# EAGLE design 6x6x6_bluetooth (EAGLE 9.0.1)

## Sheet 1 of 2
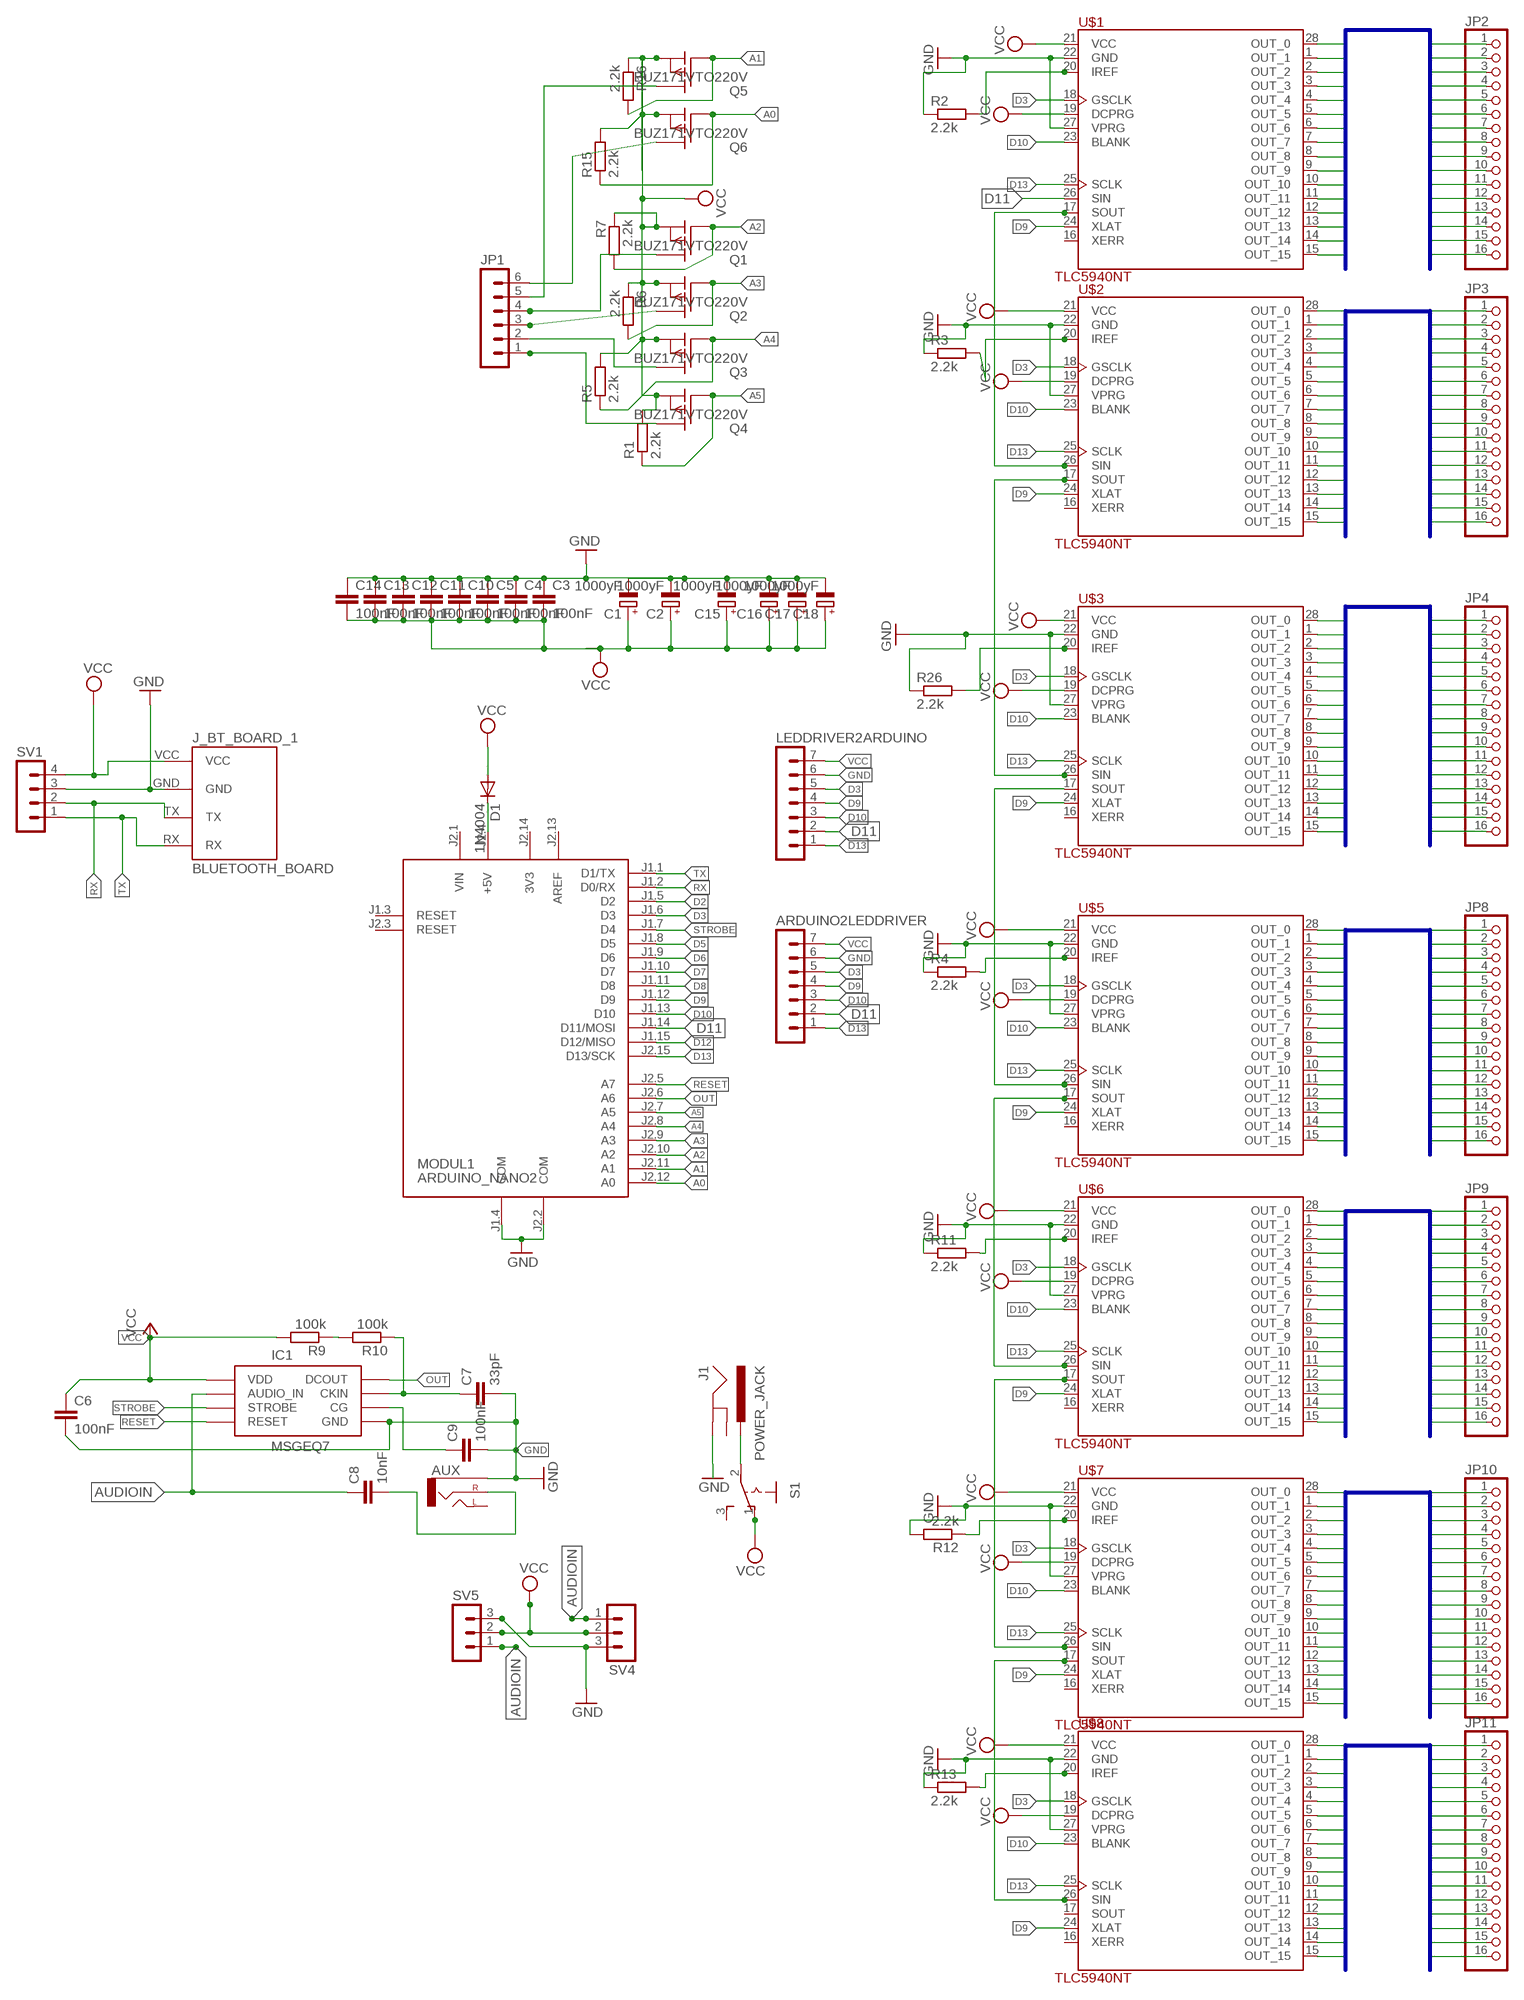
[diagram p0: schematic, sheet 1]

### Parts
ARDUINO2LEDDRIVER  MA07-1  [MA07-1]
AUX  AUDIO-JACKPTH  [AUDIO-JACK]
C1  1000yF  CPOL-EUE2.5-6  [E2,5-6]
C2  1000yF  CPOL-EUE2.5-6  [E2,5-6]
C3  100nF  C-EU025-024X044  [C025-024X044]
C4  100nF  C-EU025-024X044  [C025-024X044]
C5  100nF  C-EU025-024X044  [C025-024X044]
C6  100nF  C-EU025-025X050  [C025-025X050]
C7  33pF  C-EU025-025X050  [C025-025X050]
C8  10nF  C-EU025-025X050  [C025-025X050]
C9  100nF  C-EU025-025X050  [C025-025X050]
C10  100nF  C-EU025-024X044  [C025-024X044]
C11  100nF  C-EU025-024X044  [C025-024X044]
C12  100nF  C-EU025-024X044  [C025-024X044]
C13  100nF  C-EU025-024X044  [C025-024X044]
C14  100nF  C-EU025-024X044  [C025-024X044]
C15  1000yF  CPOL-EUE2.5-6  [E2,5-6]
C16  1000yF  CPOL-EUE2.5-6  [E2,5-6]
C17  1000yF  CPOL-EUE2.5-6  [E2,5-6]
C18  1000yF  CPOL-EUE2.5-6  [E2,5-6]
D1  1N4004  [DO41-10]
IC1  MSGEQ7DIP  [DIL08]
J1  POWER_JACK  [POWER_JACK_PTH]
J_BT_BOARD_1  BLUETOOTH_BOARD  [BT_BOARD_FOOTPRINT]
JP1  MA06-1  [MA06-1]
JP2  PINHD-1X16  [1X16]
JP3  PINHD-1X16  [1X16]
JP4  PINHD-1X16  [1X16]
JP8  PINHD-1X16  [1X16]
JP9  PINHD-1X16  [1X16]
JP10  PINHD-1X16  [1X16]
JP11  PINHD-1X16  [1X16]
LEDDRIVER2ARDUINO  MA07-1  [MA07-1]
MODUL1  ARDUINO_NANO2  [ARDUINO_NANO2]
Q1  BUZ171VTO220V  [TO220V]
Q2  BUZ171VTO220V  [TO220V]
Q3  BUZ171VTO220V  [TO220V]
Q4  BUZ171VTO220V  [TO220V]
Q5  BUZ171VTO220V  [TO220V]
Q6  BUZ171VTO220V  [TO220V]
R1  2.2k  R-EU_0204/7  [0204/7]
R2  2.2k  R-EU_0207/10  [0207/10]
R3  2.2k  R-EU_0207/10  [0207/10]
R4  2.2k  R-EU_0204/7  [0204/7]
R5  2.2k  R-EU_0204/7  [0204/7]
R6  2.2k  R-EU_0204/7  [0204/7]
R7  2.2k  R-EU_0204/7  [0204/7]
R9  100k  R-EU_0204/2V  [0204V]
R10  100k  R-EU_0204/2V  [0204V]
R11  2.2k  R-EU_0204/2V  [0204V]
R12  2.2k  R-EU_0204/2V  [0204V]
R13  2.2k  R-EU_0204/2V  [0204V]
R15  2.2k  R-EU_0204/7  [0204/7]
R16  2.2k  R-EU_0204/7  [0204/7]
R26  2.2k  R-EU_0204/5  [0204/5]
S1  255SB  [255SB]
SV1  MA04-1  [MA04-1]
SV4  MA03-1  [MA03-1]
SV5  MA03-1  [MA03-1]
U$1  TLC5940NT  [DIP-28]
U$2  TLC5940NT  [DIP-28]
U$3  TLC5940NT  [DIP-28]
U$5  TLC5940NT  [DIP-28]
U$6  TLC5940NT  [DIP-28]
U$7  TLC5940NT  [DIP-28]
U$8  TLC5940NT  [DIP-28]

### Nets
A0: MODUL1.J2.12(A0) Q6.1(G) R15.1
A1: MODUL1.J2.11(A1) Q5.1(G) R16.2
A2: MODUL1.J2.10(A2) Q1.1(G) R7.2
A3: MODUL1.J2.9(A3) Q2.1(G) R6.2
A4: MODUL1.J2.8(A4) Q3.1(G) R5.1
A5: MODUL1.J2.7(A5) Q4.1(G) R1.1
AUDIOIN: C8.1 IC1.5(AUDIO_IN) SV4.1 SV5.1
D2: MODUL1.J1.5(D2)
D3: ARDUINO2LEDDRIVER.5 LEDDRIVER2ARDUINO.5 MODUL1.J1.6(D3) U$1.18(GSCLK) U$2.18(GSCLK) U$3.18(GSCLK) U$5.18(GSCLK) U$6.18(GSCLK) U$7.18(GSCLK) U$8.18(GSCLK)
D5: MODUL1.J1.8(D5)
D6: MODUL1.J1.9(D6)
D7: MODUL1.J1.10(D7)
D8: MODUL1.J1.11(D8)
D9: ARDUINO2LEDDRIVER.4 LEDDRIVER2ARDUINO.4 MODUL1.J1.12(D9) U$1.24(XLAT) U$2.24(XLAT) U$3.24(XLAT) U$5.24(XLAT) U$6.24(XLAT) U$7.24(XLAT) U$8.24(XLAT)
D10: ARDUINO2LEDDRIVER.3 LEDDRIVER2ARDUINO.3 MODUL1.J1.13(D10) U$1.23(BLANK) U$2.23(BLANK) U$3.23(BLANK) U$5.23(BLANK) U$6.23(BLANK) U$7.23(BLANK) U$8.23(BLANK)
D11: ARDUINO2LEDDRIVER.2 LEDDRIVER2ARDUINO.2 MODUL1.J1.14(D11/MOSI) U$1.26(SIN)
D12: MODUL1.J1.15(D12/MISO)
D13: ARDUINO2LEDDRIVER.1 LEDDRIVER2ARDUINO.1 MODUL1.J2.15(D13/SCK) U$1.25(SCLK) U$2.25(SCLK) U$3.25(SCLK) U$5.25(SCLK) U$6.25(SCLK) U$7.25(SCLK) U$8.25(SCLK)
GND: ARDUINO2LEDDRIVER.6 AUX.SLEEVE C1.- C2.- C3.1 C4.1 C5.1 C6.2 C7.2 C9.2 C10.1 C11.1 C12.1 C13.1 C14.1 C15.- C16.- C17.- C18.- IC1.2(GND) J1.GND J_BT_BOARD_1.GND LEDDRIVER2ARDUINO.6 MODUL1.J1.4(COM) MODUL1.J2.2(COM) R2.1 R3.1 R4.1 R11.1 R12.2 R13.1 R26.1 SV1.3 SV4.3 SV5.3 U$1.22(GND) U$1.27(VPRG) U$2.22(GND) U$2.27(VPRG) U$3.22(GND) U$3.27(VPRG) U$5.22(GND) U$5.27(VPRG) U$6.22(GND) U$6.27(VPRG) U$7.22(GND) U$7.27(VPRG) U$8.22(GND) U$8.27(VPRG)
N$1: J1.PWR S1.2(P)
N$2: JP1.3 Q2.2(D)
N$4: JP1.1 Q4.2(D)
N$5: U$1.17(SOUT) U$2.26(SIN)
N$6: U$2.17(SOUT) U$3.26(SIN)
N$7: R26.2 U$3.20(IREF)
N$8: R3.2 U$2.20(IREF)
N$9: R2.2 U$1.20(IREF)
N$10: JP1.2 Q3.2(D)
N$11: JP1.4 Q1.2(D)
N$55: AUX.RING(RIGHT) C8.2
N$93: C9.1 IC1.6(CG)
N$94: C7.1 IC1.8(CKIN) R10.1
N$95: R9.1 R10.2
N$96: U$3.17(SOUT) U$5.26(SIN)
N$97: JP1.5 Q5.2(D)
N$98: R4.2 U$5.20(IREF)
N$99: U$5.17(SOUT) U$6.26(SIN)
N$100: U$6.17(SOUT) U$7.26(SIN)
N$101: R11.2 U$6.20(IREF)
N$102: D1.C MODUL1.J2.4(+5V)
N$103: U$7.17(SOUT) U$8.26(SIN)
N$104: R12.1 U$7.20(IREF)
N$105: JP1.6 Q6.2(D)
N$107: R13.2 U$8.20(IREF)
OUT: IC1.3(DCOUT) MODUL1.J2.6(A6)
RESET: IC1.7(RESET) MODUL1.J2.5(A7)
RX: J_BT_BOARD_1.TX MODUL1.J1.2(D0/RX) SV1.2
STROBE: IC1.4(STROBE) MODUL1.J1.7(D4)
T1OUT0: JP2.1 U$1.28(OUT_0)
T1OUT1: JP2.2 U$1.1(OUT_1)
T1OUT2: JP2.3 U$1.2(OUT_2)
T1OUT3: JP2.4 U$1.3(OUT_3)
T1OUT4: JP2.5 U$1.4(OUT_4)
T1OUT5: JP2.6 U$1.5(OUT_5)
T1OUT6: JP2.7 U$1.6(OUT_6)
T1OUT7: JP2.8 U$1.7(OUT_7)
T1OUT8: JP2.9 U$1.8(OUT_8)
T1OUT9: JP2.10 U$1.9(OUT_9)
T1OUT10: JP2.11 U$1.10(OUT_10)
T1OUT11: JP2.12 U$1.11(OUT_11)
T1OUT12: JP2.13 U$1.12(OUT_12)
T1OUT13: JP2.14 U$1.13(OUT_13)
T1OUT14: JP2.15 U$1.14(OUT_14)
T1OUT15: JP2.16 U$1.15(OUT_15)
T2OUT0: JP3.1 U$2.28(OUT_0)
T2OUT1: JP3.2 U$2.1(OUT_1)
T2OUT2: JP3.3 U$2.2(OUT_2)
T2OUT3: JP3.4 U$2.3(OUT_3)
T2OUT4: JP3.5 U$2.4(OUT_4)
T2OUT5: JP3.6 U$2.5(OUT_5)
T2OUT6: JP3.7 U$2.6(OUT_6)
T2OUT7: JP3.8 U$2.7(OUT_7)
T2OUT8: JP3.9 U$2.8(OUT_8)
T2OUT9: JP3.10 U$2.9(OUT_9)
T2OUT10: JP3.11 U$2.10(OUT_10)
T2OUT11: JP3.12 U$2.11(OUT_11)
T2OUT12: JP3.13 U$2.12(OUT_12)
T2OUT13: JP3.14 U$2.13(OUT_13)
T2OUT14: JP3.15 U$2.14(OUT_14)
T2OUT15: JP3.16 U$2.15(OUT_15)
T3OUT_0: JP4.1 U$3.28(OUT_0)
T3OUT_1: JP4.2 U$3.1(OUT_1)
T3OUT_2: JP4.3 U$3.2(OUT_2)
T3OUT_3: JP4.4 U$3.3(OUT_3)
T3OUT_4: JP4.5 U$3.4(OUT_4)
T3OUT_5: JP4.6 U$3.5(OUT_5)
T3OUT_6: JP4.7 U$3.6(OUT_6)
T3OUT_7: JP4.8 U$3.7(OUT_7)
T3OUT_8: JP4.9 U$3.8(OUT_8)
T3OUT_9: JP4.10 U$3.9(OUT_9)
T3OUT_10: JP4.11 U$3.10(OUT_10)
T3OUT_11: JP4.12 U$3.11(OUT_11)
T3OUT_12: JP4.13 U$3.12(OUT_12)
T3OUT_13: JP4.14 U$3.13(OUT_13)
T3OUT_14: JP4.15 U$3.14(OUT_14)
T3OUT_15: JP4.16 U$3.15(OUT_15)
T4OUT0: JP8.1 U$5.28(OUT_0)
T4OUT1: JP8.2 U$5.1(OUT_1)
T4OUT2: JP8.3 U$5.2(OUT_2)
T4OUT3: JP8.4 U$5.3(OUT_3)
T4OUT4: JP8.5 U$5.4(OUT_4)
T4OUT5: JP8.6 U$5.5(OUT_5)
T4OUT6: JP8.7 U$5.6(OUT_6)
T4OUT7: JP8.8 U$5.7(OUT_7)
T4OUT8: JP8.9 U$5.8(OUT_8)
T4OUT9: JP8.10 U$5.9(OUT_9)
T4OUT10: JP8.11 U$5.10(OUT_10)
T4OUT11: JP8.12 U$5.11(OUT_11)
T4OUT12: JP8.13 U$5.12(OUT_12)
T4OUT13: JP8.14 U$5.13(OUT_13)
T4OUT14: JP8.15 U$5.14(OUT_14)
T4OUT15: JP8.16 U$5.15(OUT_15)
T5OUT0: JP9.1 U$6.28(OUT_0)
T5OUT1: JP9.2 U$6.1(OUT_1)
T5OUT2: JP9.3 U$6.2(OUT_2)
T5OUT3: JP9.4 U$6.3(OUT_3)
T5OUT4: JP9.5 U$6.4(OUT_4)
T5OUT5: JP9.6 U$6.5(OUT_5)
T5OUT6: JP9.7 U$6.6(OUT_6)
T5OUT7: JP9.8 U$6.7(OUT_7)
T5OUT8: JP9.9 U$6.8(OUT_8)
T5OUT9: JP9.10 U$6.9(OUT_9)
T5OUT10: JP9.11 U$6.10(OUT_10)
T5OUT11: JP9.12 U$6.11(OUT_11)
T5OUT12: JP9.13 U$6.12(OUT_12)
T5OUT13: JP9.14 U$6.13(OUT_13)
T5OUT14: JP9.15 U$6.14(OUT_14)
T5OUT15: JP9.16 U$6.15(OUT_15)
T6OUT0: JP10.1 U$7.28(OUT_0)
T6OUT1: JP10.2 U$7.1(OUT_1)
T6OUT2: JP10.3 U$7.2(OUT_2)
T6OUT3: JP10.4 U$7.3(OUT_3)
T6OUT4: JP10.5 U$7.4(OUT_4)
T6OUT5: JP10.6 U$7.5(OUT_5)
T6OUT6: JP10.7 U$7.6(OUT_6)
T6OUT7: JP10.8 U$7.7(OUT_7)
T6OUT8: JP10.9 U$7.8(OUT_8)
T6OUT9: JP10.10 U$7.9(OUT_9)
T6OUT10: JP10.11 U$7.10(OUT_10)
T6OUT11: JP10.12 U$7.11(OUT_11)
T6OUT12: JP10.13 U$7.12(OUT_12)
T6OUT13: JP10.14 U$7.13(OUT_13)
T6OUT14: JP10.15 U$7.14(OUT_14)
T6OUT15: JP10.16 U$7.15(OUT_15)
T7OUT0: JP11.1 U$8.28(OUT_0)
T7OUT1: JP11.2 U$8.1(OUT_1)
T7OUT2: JP11.3 U$8.2(OUT_2)
T7OUT3: JP11.4 U$8.3(OUT_3)
T7OUT4: JP11.5 U$8.4(OUT_4)
T7OUT5: JP11.6 U$8.5(OUT_5)
T7OUT6: JP11.7 U$8.6(OUT_6)
T7OUT7: JP11.8 U$8.7(OUT_7)
T7OUT8: JP11.9 U$8.8(OUT_8)
T7OUT9: JP11.10 U$8.9(OUT_9)
T7OUT10: JP11.11 U$8.10(OUT_10)
T7OUT11: JP11.12 U$8.11(OUT_11)
T7OUT12: JP11.13 U$8.12(OUT_12)
T7OUT13: JP11.14 U$8.13(OUT_13)
T7OUT14: JP11.15 U$8.14(OUT_14)
T7OUT15: JP11.16 U$8.15(OUT_15)
TX: J_BT_BOARD_1.RX MODUL1.J1.1(D1/TX) SV1.1
VCC: ARDUINO2LEDDRIVER.7 C1.+ C2.+ C3.2 C4.2 C5.2 C6.1 C10.2 C11.2 C12.2 C13.2 C14.2 C15.+ C16.+ C17.+ C18.+ D1.A IC1.1(VDD) J_BT_BOARD_1.VCC LEDDRIVER2ARDUINO.7 Q1.3(S) Q2.3(S) Q3.3(S) Q4.3(S) Q5.3(S) Q6.3(S) R1.2 R5.2 R6.1 R7.1 R9.2 R15.2 R16.1 S1.1(O) SV1.4 SV4.2 SV5.2 U$1.19(DCPRG) U$1.21(VCC) U$2.19(DCPRG) U$2.21(VCC) U$3.19(DCPRG) U$3.21(VCC) U$5.19(DCPRG) U$6.19(DCPRG) U$6.21(VCC) U$7.19(DCPRG) U$7.21(VCC) U$8.19(DCPRG) U$8.21(VCC)
Unconnected: AUX.TIP(LEFT) J1.GNDBREAK MODUL1.J1.3(RESET) MODUL1.J2.3(RESET) S1.3(S) U$1.16(XERR) U$2.16(XERR) U$3.16(XERR) U$5.16(XERR) U$6.16(XERR) U$7.16(XERR) U$8.16(XERR) U$8.17(SOUT)

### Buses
T3OUT_[0..15]
T2OUT[0..15]
T1OUT[0..15]
T4OUT[0..15]
T5OUT[0..15]
T6OUT[0..15]
T7OUT[0..15]

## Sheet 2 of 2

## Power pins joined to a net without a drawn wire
3V3: MODUL1.J2.14(3V3)
AREF: MODUL1.J2.13(AREF)
VCC: U$5.21(VCC)
VIN: MODUL1.J2.1(VIN)

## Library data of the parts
ARDUINO2LEDDRIVER LEDDRIVER2ARDUINO = con-lstb:MA07-1: PIN HEADER; OC_FARNELL: unknown; OC_NEWARK: unknown
AUX = connector:AUDIO-JACK: 3.5mm Audio Jack Simple 3.5mm common PCB mount audio jack.; DIGIKEY: CP1-3524N-ND
C1 C2 C15-C18 = resistor:CPOL-EU: POLARIZED CAPACITOR, European symbol
C3-C14 = resistor:C-EU: CAPACITOR, European symbol
D1 = diode:1N4004: DIODE
IC1 = msgeq7:MSGEQ7: 7-band graphic equalizer
J1 = SparkFun-Connectors:POWER_JACK: Power Jack Connector This is the standard 5.5mm barrel jack for power. The PTH is the most common, proven, reliable, footprint. The Slot footprint only works if the mill layer is transmitted to the PCB fab house so be warned. Here are the connectors we sell at SparkFun: DC Barrel Power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; PROD_ID: CONN-08197
J_BT_BOARD_1 = Bluetooth HC-05:BLUETOOTH_BOARD: Bluetooth Board V1.05
JP1 = con-lstb:MA06-1: PIN HEADER; OC_FARNELL: unknown; OC_NEWARK: unknown
JP2-JP4 JP8-JP11 = pinhead:PINHD-1X16: PIN HEADER
MODUL1 = arduino:ARDUINO_NANO2: Arduino Nano2 Auto generated by modulcreator.ulp \;; ANZAHL: 2; MODUL: TRUE; STECKX0: -76200; STECKX1: 76200; STECKY0: 177800; STECKY1: 177800
Q1-Q6 = transistor-fet:BUZ171V: P-Channel Enhancement MOSFET -50V; 7A; 0,4Ohm
R1-R7 R9-R13 R15 R16 R26 = resistor:R-EU_: RESISTOR, European symbol
S1 = switch:255SB: SLIDING SWITCH Distributor Buerklin, 11G810
SV1 = con-lstb:MA04-1: PIN HEADER; OC_FARNELL: unknown; OC_NEWARK: unknown
SV4 SV5 = con-lstb:MA03-1: PIN HEADER; OC_FARNELL: unknown; OC_NEWARK: unknown
U$1-U$3 U$5-U$8 = tlc5940:TLC5940

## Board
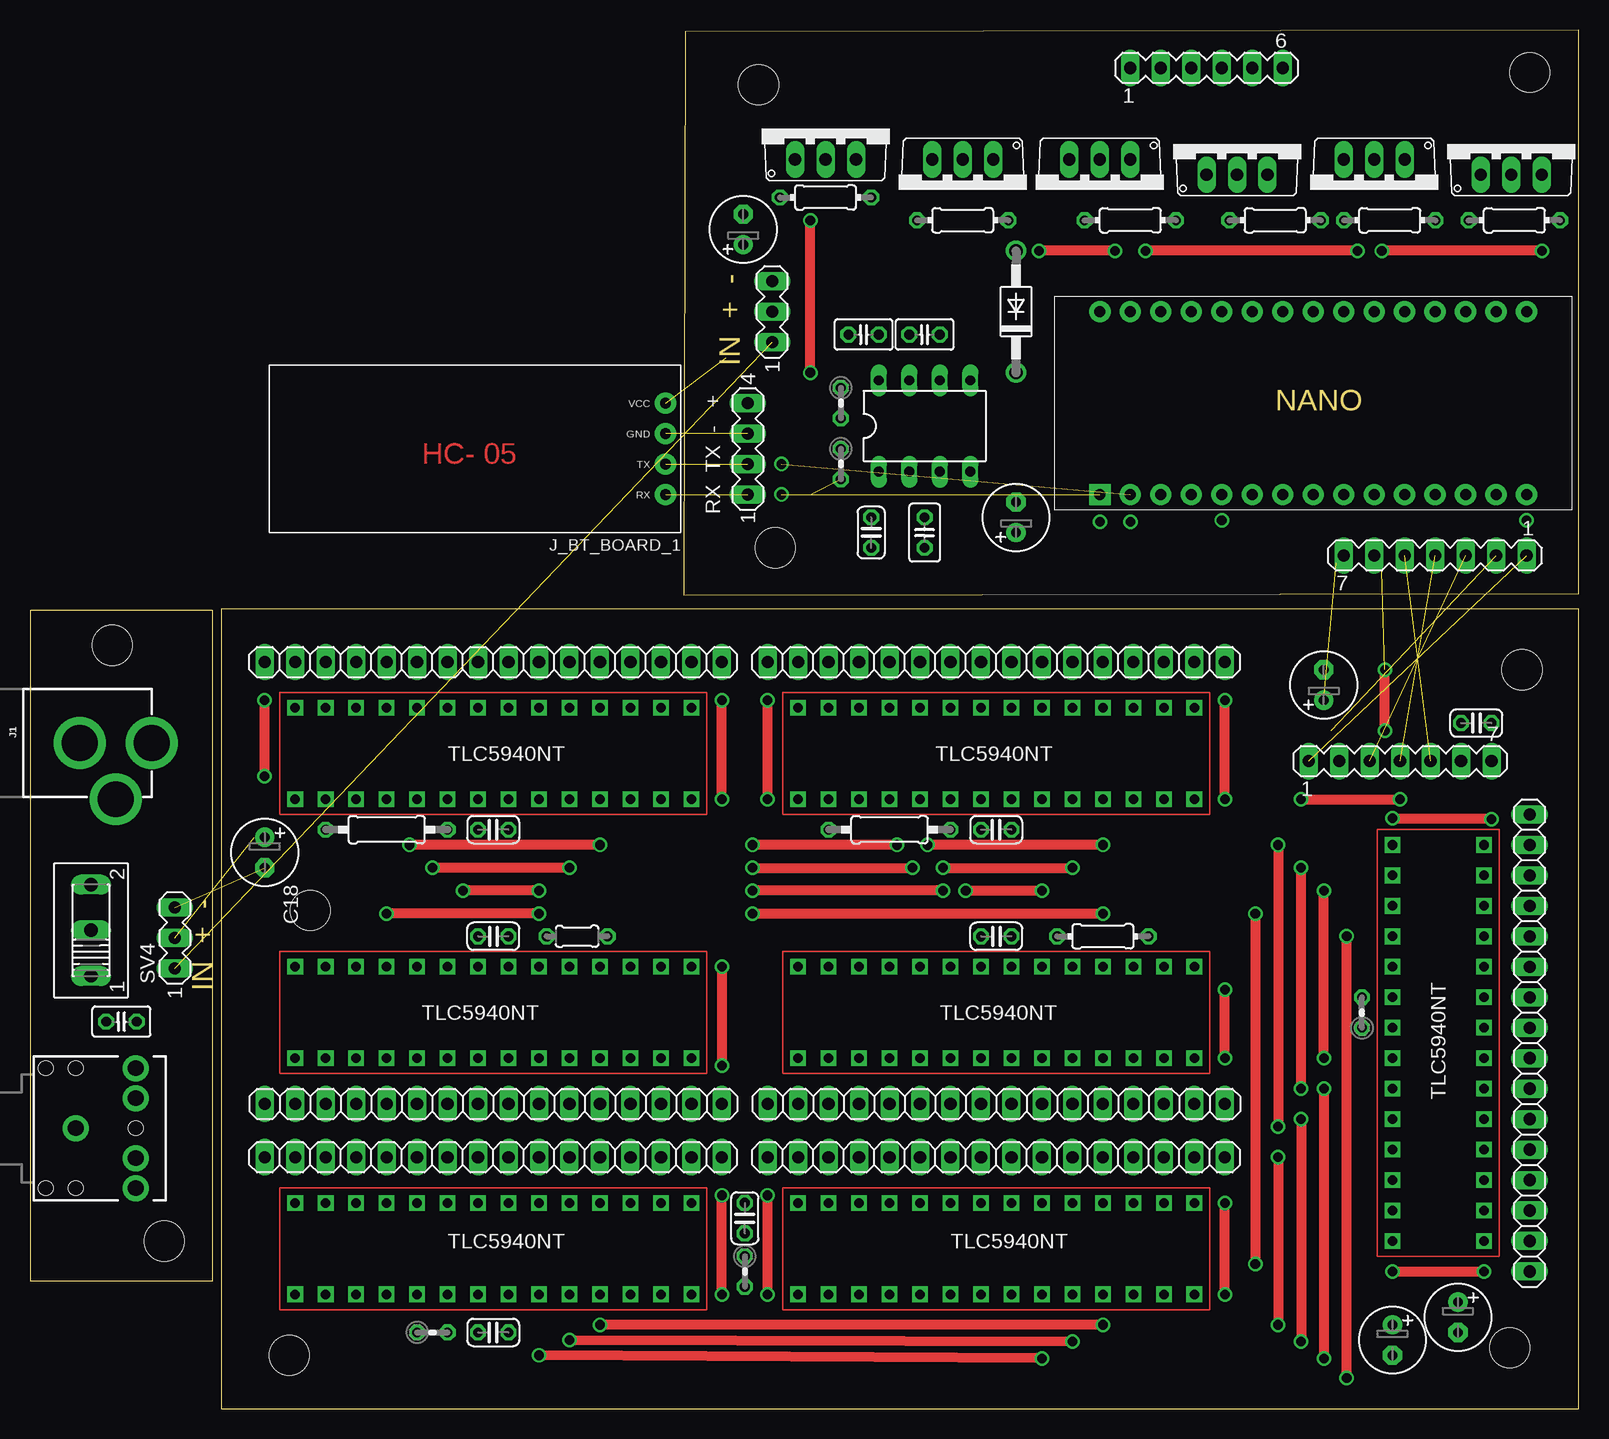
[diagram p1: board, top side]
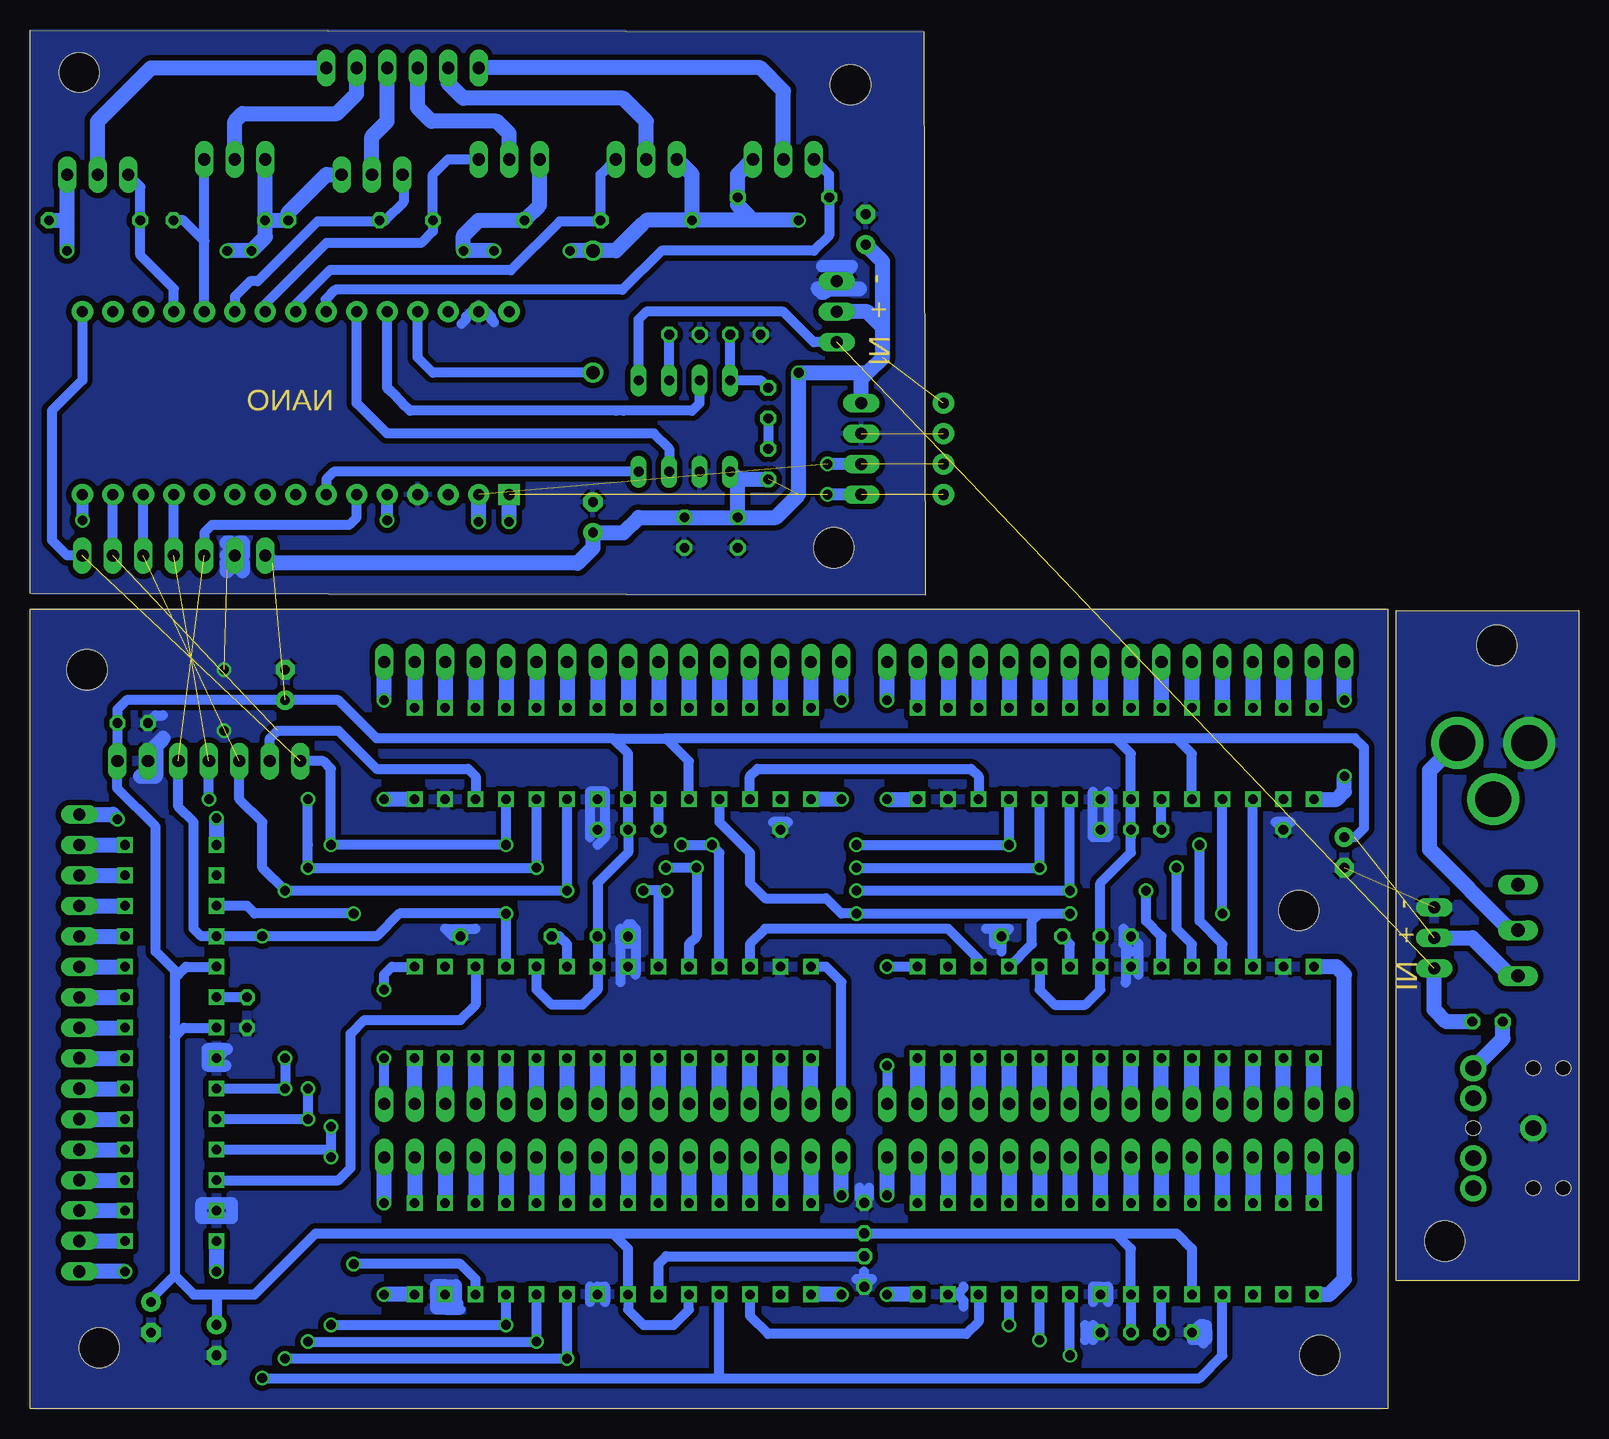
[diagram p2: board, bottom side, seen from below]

Size 129.08 x 114.93 mm. Coordinates in mm from the lower left corner, seen from the top.
Outline: 54.48,67.82 129.08,67.95 129.08,114.93 54.61,114.8 54.48,67.82
Outline: 15.93,0 129.08,0 129.08,66.67 15.93,66.67 15.93,0
Outline: 0,66.55 0,10.67 15.24,10.67 15.24,66.55 0,66.55
Copper layers (1*16): Top 0.035mm / dielectric 1.5mm / Bottom 0.035mm
Design rules "default *": minimum track width 32mil, minimum drill 0.8mm, track to track 18mil, track to pad 8mil, pad to pad 8mil, via to via 8mil, smd to smd 8mil, copper to edge 0mil, drill to drill 8mil, minimum pad ring 10mil, minimum via ring 8mil, stop-mask expansion 4mil, vias tented up to drill 0mil, thermal gap 10mil
Holes 3.33 mm at 23.37,41.53 21.59,4.45 123.32,5.08 124.33,61.59 62.1,71.75 60.71,110.36 11.18,13.97 6.86,63.63
Holes 3.3 mm at 124.97,111.38

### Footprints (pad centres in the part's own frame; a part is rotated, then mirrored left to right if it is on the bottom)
MA07-1 = drill 1.016 long: 1 -7.62,0; 2 -5.08,0; 3 -2.54,0; 4 0,0; 5 2.54,0; 6 5.08,0; 7 7.62,0
AUDIO-JACK = drill 1.3 pad 2.184: RING 5,5; RSH 5,2.5; SLEEVE 0,0; TIP 5,-5; TSH 5,-2.5 | hole 1.2: 0,5; -2.5,5; -2.5,-5; 0,-5; 5,0
E2,5-6 = drill 0.813 pad 1.6: + -1.27,0 | drill 0.813 pad 1.6 octagon: - 1.27,0
C025-024X044 = drill 0.813 octagon: 1 -1.27,0; 2 1.27,0
C025-025X050 = drill 0.813 octagon: 1 -1.27,0; 2 1.27,0
DO41-10 = drill 1.118: A 5.08,0; C -5.08,0
DIL08 = drill 0.813 long: 1 -3.81,-3.81; 2 -1.27,-3.81; 3 1.27,-3.81; 4 3.81,-3.81; 5 3.81,3.81; 6 1.27,3.81; 7 -1.27,3.81; 8 -3.81,3.81
POWER_JACK_PTH = drill 2.997 pad 4.318: GND 0,7.7; GNDBREAK 4.7,10.7; PWR 0,13.7
BT_BOARD_FOOTPRINT = drill 0.9 pad 1.778: GND -16.51,-1.27; RX -16.51,3.81; TX -16.51,1.27; VCC -16.51,-3.81
MA06-1 = drill 1.016 long: 1 -6.35,0; 2 -3.81,0; 3 -1.27,0; 4 1.27,0; 5 3.81,0; 6 6.35,0
1X16 = drill 1.016 long: 1 -19.05,0; 2 -16.51,0; 3 -13.97,0; 4 -11.43,0; 5 -8.89,0; 6 -6.35,0; 7 -3.81,0; 8 -1.27,0; 9 1.27,0; 10 3.81,0; 11 6.35,0; 12 8.89,0; 13 11.43,0; 14 13.97,0; 15 16.51,0; 16 19.05,0
ARDUINO_NANO2 = drill 0.914 pad 1.778 square: J1.1 -7.62,17.78 | drill 0.914 pad 1.778: J1.2 -7.62,15.24; J1.3 -7.62,12.7; J1.4 -7.62,10.16; J1.5 -7.62,7.62; J1.6 -7.62,5.08; J1.7 -7.62,2.54; J1.8 -7.62,0; J1.9 -7.62,-2.54; J1.10 -7.62,-5.08; J1.11 -7.62,-7.62; J1.12 -7.62,-10.16; J1.13 -7.62,-12.7; J1.14 -7.62,-15.24; J1.15 -7.62,-17.78; J2.1 7.62,17.78; J2.2 7.62,15.24; J2.3 7.62,12.7; J2.4 7.62,10.16; J2.5 7.62,7.62; J2.6 7.62,5.08; J2.7 7.62,2.54; J2.8 7.62,0; J2.9 7.62,-2.54; J2.10 7.62,-5.08; J2.11 7.62,-7.62; J2.12 7.62,-10.16; J2.13 7.62,-12.7; J2.14 7.62,-15.24; J2.15 7.62,-17.78
TO220V = drill 1.016 long: 1 -2.54,-2.54; 2 0,-2.54; 3 2.54,-2.54
0204/7 = drill 0.813 octagon: 1 -3.81,0; 2 3.81,0
0207/10 = drill 0.813 octagon: 1 -5.08,0; 2 5.08,0
0204V = drill 0.813 octagon: 1 -1.27,0; 2 1.27,0
0204/5 = drill 0.813 octagon: 1 -2.54,0; 2 2.54,0
255SB = drill 1.118 long: 1 -3.81,0; 2 0,0; 3 3.81,0
MA04-1 = drill 1.016 long: 1 -3.81,0; 2 -1.27,0; 3 1.27,0; 4 3.81,0
MA03-1 = drill 1.016 long: 1 -2.54,0; 2 0,0; 3 2.54,0
DIP-28 = drill 0.8 square: 1 -3.81,-1.27; 2 -3.81,-3.81; 3 -3.81,-6.35; 4 -3.81,-8.89; 5 -3.81,-11.43; 6 -3.81,-13.97; 7 -3.81,-16.51; 8 -3.81,-19.05; 9 -3.81,-21.59; 10 -3.81,-24.13; 11 -3.81,-26.67; 12 -3.81,-29.21; 13 -3.81,-31.75; 14 -3.81,-34.29; 15 3.81,-34.29; 16 3.81,-31.75; 17 3.81,-29.21; 18 3.81,-26.67; 19 3.81,-24.13; 20 3.81,-21.59; 21 3.81,-19.05; 22 3.81,-16.51; 23 3.81,-13.97; 24 3.81,-11.43; 25 3.81,-8.89; 26 3.81,-6.35; 27 3.81,-3.81; 28 3.81,-1.27

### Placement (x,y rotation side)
ARDUINO2LEDDRIVER  114.17,53.98 0 top
AUX  3.81,23.37 0 top
C1  82.17,74.3 90 top
C2  107.82,60.33 90 top
C3  38.61,6.35 180 top
C4  80.52,48.26 180 top
C5  38.61,39.37 0 top
C6  74.55,73.03 270 top
C7  69.47,89.53 180 top
C8  7.62,32.26 180 top
C9  74.55,89.53 180 top
C10  70.1,73.03 90 top
C11  38.61,48.26 180 top
C12  59.56,15.88 270 top
C13  120.52,57.15 0 top
C14  80.52,39.37 0 top
C15  113.54,5.72 270 top
C16  119,7.62 270 top
C17  59.44,98.3 90 top
C18  19.56,46.36 270 top
D1  82.17,91.44 90 top
IC1  74.55,81.91 0 top
J1  -3.56,55.5 270 top
J_BT_BOARD_1  36.45,80.01 180 top
JP1  98.04,111.76 0 top
JP2  80.52,62.23 180 top
JP3  38.61,62.23 180 top
JP4  38.61,25.4 0 top
JP8  80.52,25.4 0 top
JP9  124.97,30.48 90 top
JP10  80.52,20.95 180 top
JP11  38.61,20.95 180 top
LEDDRIVER2ARDUINO  117.09,71.12 180 top
MODUL1  106.93,83.82 90 top
Q1  100.58,105.41 0 top
Q2  89.15,101.6 180 top
Q3  77.72,101.6 180 top
Q4  66.29,106.68 0 top
Q5  112.01,101.6 180 top
Q6  123.44,105.41 0 top
R1  66.29,100.97 0 top
R2  71.63,48.26 0 top
R3  29.72,48.26 0 top
R4  89.41,39.37 180 top
R5  77.72,99.06 180 top
R6  91.69,99.06 0 top
R7  103.76,99.06 180 top
R9  67.56,78.74 270 top
R10  67.56,83.82 270 top
R11  111,33.02 90 top
R12  59.56,11.43 270 top
R13  33.53,6.35 0 top
R15  123.7,99.06 0 top
R16  113.31,99.06 0 top
R26  45.59,39.37 180 top
S1  5.08,39.88 90 top
SV1  59.82,80.01 90 top
SV4  12.06,39.24 90 top
SV5  61.85,91.44 90 top
U$1  98.3,54.61 270 top
U$2  56.39,54.61 270 top
U$3  20.83,33.02 90 top
U$5  62.74,33.02 90 top
U$6  117.35,12.7 180 top
U$7  98.3,13.34 270 top
U$8  56.39,13.34 270 top

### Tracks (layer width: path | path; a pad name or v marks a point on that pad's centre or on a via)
A0
  Bottom 0.813: MODUL1.J2.12 117.09,93.34 119.89,96.14 R15.1 119.89,101.85 Q6.1
A1
  Bottom 0.813: 114.55,97.32 Q5.1 | MODUL1.J2.11 114.55,97.32 | R16.2 116.29,99.06 114.55,97.32
A2
  Bottom 0.813: MODUL1.J2.10 112.01,92.71 110.74,93.98 110.11,93.98 105.14,98.95 100.06,98.95 R7.2 99.46,99.06 97.95,100.57 97.95,102.78 Q1.1
A3
  Bottom 0.813: Q2.1 94.23,104.14 95.5,102.87 R6.2 95.51,98.13 96.49,97.16 104.39,97.16 109.47,92.08 MODUL1.J2.9
A4
  Bottom 0.813: Q3.1 81.53,102.87 R5.1 81.65,98.95 84.95,98.95 89.01,94.88 104.12,94.88 106.93,92.08 MODUL1.J2.8
A5
  Bottom 0.813: Q4.1 62.48,102.87 R1.1 62.48,97.79 63.75,96.52 76.45,96.52 79.71,93.26 103.64,93.26 104.45,92.45 104.39,92.39 MODUL1.J2.7
AUDIOIN  (1 unrouted)
  Bottom 0.813: IC1.5 78.36,90.81 77.72,91.44 66.29,91.44 63.75,88.9 SV5.1
  Bottom 1.27: 12.06,34.8 SV4.1 12.06,33.27 11.05,32.26 C8.1
D2  (via drill 0.8)
  Bottom 1.016: v99.31,74.04 MODUL1.J1.5
D3  (via drill 0.8)  (1 unrouted)
  Top 0.813: v42.42,41.28 v29.72,41.28 | v60.2,41.28 v89.41,41.28 | v109.73,2.54 v109.73,39.37
  Bottom 0.813: U$5.18 v89.41,41.28 98.3,41.28 100.2,39.37 v109.73,39.37 U$6.18 114.81,39.37 115.44,40.01 115.44,48.9 116.71,50.16 ARDUINO2LEDDRIVER.5 | 44.96,41.28 v60.2,41.28 61.47,41.28 62.74,42.55 67.82,42.55 69.09,43.81 69.09,46.36 71.63,48.9 U$1.18 | 44.96,41.28 v42.42,41.28 | U$8.18 29.72,4.45 31.62,2.54 71.92,2.54 | v29.72,41.28 U$2.18 | U$3.18 45.59,38.73 45.59,40.64 44.96,41.28 | MODUL1.J1.6 101.85,74.3 102.49,73.66 113.92,73.66 114.55,73.03 LEDDRIVER2ARDUINO.5 | v109.73,2.54 71.92,2.54 | 71.92,2.54 71.63,2.83 U$7.18
D9  (via drill 0.8)  (1 unrouted)
  Top 0.813: v60.2,45.09 v73.53,45.09 | v44.96,45.09 v33.53,45.09 | v76.07,45.09 v86.87,45.09 | v105.92,26.67 v105.92,45.09 | v105.92,24.13 v105.92,5.59 | v86.87,5.59 v44.96,5.72 | v105.92,50.8 v114.17,50.8
  Bottom 0.813: LEDDRIVER2ARDUINO.4 MODUL1.J1.12 | v60.2,45.09 v44.96,45.09 U$2.24 | v76.07,45.09 v73.53,45.09 73.53,39.37 74.17,38.73 U$5.24 | v105.92,45.09 v86.87,45.09 U$1.24 | v105.92,45.09 105.92,46.99 | v105.92,45.09 v105.92,50.8 | v105.92,26.67 v105.92,24.13 U$6.24 | v105.92,5.59 v86.87,5.59 U$7.24 | v114.17,50.8 ARDUINO2LEDDRIVER.4 | v44.96,5.72 U$8.24 | U$3.24 32.26,38.73 33.53,40.01 v33.53,45.09
D10  (via drill 0.8)  (1 unrouted)
  Top 0.813: v42.42,43.18 v36.07,43.18 | v77.98,43.18 v84.33,43.18 | v107.82,29.21 v107.82,43.18 | v107.82,26.67 v107.82,4.19 | v84.33,4.19 v42.42,4.45 | v76.07,43.18 v60.2,43.18
  Bottom 0.813: LEDDRIVER2ARDUINO.3 MODUL1.J1.13 | v60.2,43.18 v42.42,43.18 U$2.23 | v107.82,29.21 v107.82,26.67 U$6.23 | v107.82,4.19 v84.33,4.19 U$7.23 | v76.07,43.18 76.71,43.18 | 76.71,43.18 v77.98,43.18 | ARDUINO2LEDDRIVER.3 111.63,50.8 109.73,48.9 109.73,45.09 v107.82,43.18 v84.33,43.18 U$1.23 | v42.42,4.45 U$8.23 | v36.07,43.18 36.07,40.64 34.8,39.37 U$3.23 | U$5.23 76.71,43.18
D11  (1 unrouted)
  Bottom 0.813: ARDUINO2LEDDRIVER.2 109.09,55.88 108.46,56.52 103.38,56.52 100.2,53.34 92.58,53.34 91.95,52.7 U$1.26 | LEDDRIVER2ARDUINO.2 MODUL1.J1.14
D12  (via drill 0.8)
  Bottom 1.016: MODUL1.J1.15 v124.71,74.04
D13  (via drill 0.8)  (1 unrouted)
  Top 0.813: v104.01,46.99 v104.01,23.49 | v104.01,20.95 v104.01,6.98 | v89.41,6.98 v47.5,6.98 | v89.41,46.99 v74.8,46.99 | v72.26,46.99 v60.2,46.99 | v47.5,46.99 v31.62,46.99
  Bottom 0.813: LEDDRIVER2ARDUINO.1 125.98,71.12 127.25,72.39 127.25,83.19 124.71,85.72 MODUL1.J2.15 | ARDUINO2LEDDRIVER.1 104.65,53.98 104.01,53.34 v104.01,46.99 v89.41,46.99 U$1.25 | v104.01,23.49 104.01,21.59 | 104.01,21.59 U$6.25 | 104.01,21.59 v104.01,20.95 | v104.01,6.98 v89.41,6.98 U$7.25 | v47.5,6.98 U$8.25 | v74.8,46.99 v72.26,46.99 71.63,46.36 U$5.25 | v60.2,46.99 v47.5,46.99 U$2.25 | U$3.25 29.72,38.73 31.62,40.64 v31.62,46.99
GND  (via drill 0.8)  (3 unrouted)
  Top 0.813: v112.9,56.52 v112.9,61.59
  Bottom 0.813: 59.56,10.8 R12.2 58.93,10.8 59.56,10.8 | 59.56,10.8 59.56,11.43 | 81.15,48.9 81.15,51.44 82.42,51.44 82.42,47.62 | C4.1 81.15,48.9 | 81.15,48.9 81.15,47.62 81.79,46.99 | R2.1 65.91,48.9 67.18,48.9 | U$2.22 39.24,51.44 39.24,47.62 40.51,47.62 40.51,51.44 | R3.1 24,48.9 25.27,48.9 | C5.1 37.97,40.01 37.97,38.73 37.34,38.1 | U$3.22 36.7,36.2 36.7,38.73 C5.1 | C5.1 37.79,38.92 37.79,35.49 | R26.1 47.5,40.01 48.77,40.01 | 48.77,40.01 49.4,40.01 | 48.13,38.1 48.13,38.73 48.77,38.73 48.77,40.01 | C14.1 79.23,39.39 79.23,40.37 78.97,40.37 78.61,40.01 78.61,38.73 | 78.61,38.73 79.88,38.73 | 79.88,38.73 79.88,40.01 | 78.61,38.73 78.61,36.2 | 79.88,38.73 79.88,35.56 | R4.1 93.85,39.37 94.49,40.01 91.95,40.01 | 81.15,8.89 81.15,10.16 81.79,10.16 U$7.22 82.42,10.16 82.42,8.89 | 59.56,10.8 60.2,10.8 | 59.16,18.41 59.16,17.55 C12.1 59.97,17.55 59.97,18.41 | C3.1 40.51,6.98 40.51,6.35 | 40.51,6.35 40.51,5.72 | 40.51,6.35 41.15,6.98 41.15,5.72 | U$8.22 39.88,10.16 | 39.88,10.16 39.24,10.16 39.24,8.89 | 39.88,10.16 40.51,10.16 40.51,8.89 | R13.1 31.56,7.05 31.29,7.05 31.29,6.24 | 31.29,6.24 31.29,5.42 31.58,5.72 32.26,5.72 | 31.29,6.24 30.99,6.54 | 30.99,6.54 30.99,6.98 | 30.99,6.54 30.99,5.72 | C13.1 118.62,57.79 117.98,57.79 | 93.22,8.26 94.49,8.26 94.49,8.36 U$7.27 | 51.82,9.52 51.31,10.03 51.31,10.05 51.3,10.06 51.3,10.16 | U$8.27 51.82,9.52 | 51.82,9.52 51.31,9.02 51.31,8.51 | 90.4,90.57 90.65,90.82 90.65,91.03 91.06,91.44 MODUL1.J2.2 92.33,91.44 92.73,91.03 92.73,90.82 93.11,90.44
  Bottom 1.016: U$7.27 94.49,10.29 | 94.49,10.29 93.6,10.29 93.6,8.89 93.47,8.76 | 94.49,10.29 95.25,10.29 95.25,8.38 95.23,8.36 94.49,8.36 | U$6.22 112.78,29.97 | 112.78,29.97 112.65,29.97 | 112.78,29.97 114.3,29.97 114.3,28.58 112.78,28.58 | U$6.27 113.54,17.15 | 113.54,17.15 112.27,17.15 112.27,15.88 114.81,15.88 114.81,17.15 113.54,17.15 | 63.1,95.23 63.08,95.25 60.58,95.25 SV5.3 62.92,92.91 63.12,92.91 63.5,93.29 63.5,93.47
  Bottom 1.27: 118.62,52.7 119.25,53.34 ARDUINO2LEDDRIVER.6 119.25,54.61 118.62,55.25 | 118.62,52.7 119.89,52.7 | LEDDRIVER2ARDUINO.6 111.38,70.48 111.38,69.85 | LEDDRIVER2ARDUINO.6 112.65,70.48 112.65,69.85 | 112.01,71.75 112.42,72.16 112.65,72.16 | LEDDRIVER2ARDUINO.6 112.01,71.75 | 112.01,71.75 111.61,72.16 111.38,72.16 111.38,71.12 112.65,71.12 | 62.48,93.34 59.94,93.34 | 118.62,55.25 117.98,55.88 | 118.62,55.25 118.62,52.7 | C14.1
  pour Bottom: 54.61,67.95 54.74,114.68 128.91,114.81 128.91,68.07
  pour Bottom: 16.26,66.29 128.78,66.29 128.78,0.38 16.38,0.38
  pour Bottom: 0.38,66.17 0.38,11.05 14.86,11.05 14.86,66.17
N$1
  Bottom 1.27: J1.PWR 12.45,53.2 12.45,46.61 5.71,39.88 S1.2
N$2
  Bottom 1.27: Q2.2 89.15,106.3 90.17,107.31 95.63,107.31 96.77,108.46 JP1.3
N$4
  Bottom 1.27: Q4.2 66.29,109.86 68.2,111.76 JP1.1
N$5
  Bottom 0.813: U$1.17 69.09,52.7 68.45,53.34 50.67,53.34 50.04,52.7 U$2.26
N$6
  Bottom 0.813: U$3.26 U$2.17
N$7
  Bottom 0.813: U$3.20 42.42,38.73 R26.2
N$8
  Bottom 0.813: 34.8,50.16 U$2.20 R3.2
N$9
  Bottom 0.813: R2.2 U$1.20
N$10
  Bottom 0.813: 86.61,109.22 92.96,109.22
  Bottom 1.27: Q3.2 77.72,107.31 79.63,109.22 92.96,109.22 94.23,110.49 JP1.2
N$11
  Bottom 1.27: Q1.2 100.58,106.05 99.31,107.31 JP1.4
N$55
  Bottom 1.27: AUX.RING 6.35,30.83 C8.2
N$93
  Bottom 0.813: IC1.6 C9.1
N$94
  Bottom 0.813: C7.1 IC1.8 68.2,85.72 R10.1
N$95
  Bottom 0.813: R10.2 R9.1
N$96
  Bottom 0.813: U$5.26 69.09,38.73 67.82,40.01 52.58,40.01 50.04,37.47 U$3.17
N$97
  Bottom 1.27: Q5.2 112.01,107.31 111.38,107.95 103.51,107.95 101.85,109.6 JP1.5
N$98
  Bottom 0.813: U$5.20 84.33,38.73 84.96,39.37 R4.2
N$99
  Bottom 0.813: U$5.17 91.95,33.66 93.22,32.39 101.22,32.39 102.36,31.24 102.36,20.07 103.38,19.05 U$6.26
N$100  (via drill 0.8)
  Top 0.813: v102.11,41.28 v102.11,12.06
  Bottom 0.813: U$7.26 91.95,10.8 93.22,12.06 v102.11,12.06 | U$6.17 111,41.91 110.36,41.28 v102.11,41.28
N$101
  Bottom 0.813: R11.2 U$6.20
N$102
  Bottom 0.813: MODUL1.J2.4 96.77,87.63 95.5,86.36 D1.C
N$103
  Bottom 0.813: U$8.26 50.04,7.24 51.05,6.22 67.56,6.22 69.09,7.75 U$7.17
N$104
  Bottom 0.813: R12.1 76.07,12.7 76.71,12.06 U$7.20
N$105
  Bottom 1.27: Q6.2 123.44,107.31 119,111.76 JP1.6
N$107
  Bottom 0.813: R13.2 U$8.20
OUT
  Bottom 0.813: IC1.3 75.82,80.01 77.09,81.28 99.31,81.28 101.85,83.82 MODUL1.J2.6
RESET
  Bottom 0.813: IC1.7 73.28,83.82 73.91,83.19 79.63,83.19 80.26,83.19 97.41,83.19 98.04,83.82 99,84.77 99.31,85.09 MODUL1.J2.5
RX  (via drill 0.8)  (2 unrouted)
  Bottom 1.016: SV1.2 v62.61,78.74
  Bottom 1.27: v91.69,73.91 MODUL1.J1.2
STROBE
  Bottom 0.813: MODUL1.J1.7 104.39,77.47 103.76,78.11 IC1.4
T1OUT0  (via drill 0.8)
  Top 0.813: v99.57,50.8 v99.57,59.05
  Bottom 1.27: U$1.28 v99.57,50.8 | v99.57,59.05 JP2.1
T1OUT1
  Bottom 1.27: JP2.2 U$1.1
T1OUT2
  Bottom 1.27: JP2.3 U$1.2
T1OUT3
  Bottom 1.27: JP2.4 U$1.3
T1OUT4
  Bottom 1.27: JP2.5 U$1.4
T1OUT5
  Bottom 1.27: JP2.6 U$1.5
T1OUT6
  Bottom 1.27: JP2.7 U$1.6
T1OUT7
  Bottom 1.27: JP2.8 U$1.7
T1OUT8
  Bottom 1.27: JP2.9 U$1.8
T1OUT9
  Bottom 1.27: JP2.10 U$1.9
T1OUT10
  Bottom 1.27: JP2.11 U$1.10
T1OUT11
  Bottom 1.27: JP2.12 U$1.11
T1OUT12
  Bottom 1.27: JP2.13 U$1.12
T1OUT13
  Bottom 1.27: JP2.14 U$1.13
T1OUT14
  Bottom 1.27: JP2.15 U$1.14
T1OUT15  (via drill 0.8)
  Top 0.813: v61.47,50.8 v61.47,59.05
  Bottom 1.27: v61.47,59.05 JP2.16 | v61.47,50.8 U$1.15
T2OUT0  (via drill 0.8)
  Top 0.813: v57.66,50.8 v57.66,59.05
  Bottom 1.27: v57.66,50.8 U$2.28 | v57.66,59.05 JP3.1
T2OUT1
  Bottom 1.27: JP3.2 U$2.1
T2OUT2
  Bottom 1.27: JP3.3 U$2.2
T2OUT3
  Bottom 1.27: JP3.4 U$2.3
T2OUT4
  Bottom 1.27: JP3.5 U$2.4
T2OUT5
  Bottom 1.27: JP3.6 U$2.5
T2OUT6
  Bottom 1.27: JP3.7 U$2.6
T2OUT7
  Bottom 1.27: JP3.8 U$2.7
T2OUT8
  Bottom 1.27: JP3.9 U$2.8
T2OUT9
  Bottom 1.27: JP3.10 U$2.9
T2OUT10
  Bottom 1.27: JP3.11 U$2.10
T2OUT11
  Bottom 1.27: JP3.12 U$2.11
T2OUT12
  Bottom 1.27: JP3.13 U$2.12
T2OUT13
  Bottom 1.27: JP3.14 U$2.13
T2OUT14
  Bottom 1.27: JP3.15 U$2.14
T2OUT15  (via drill 0.8)
  Top 0.813: v19.56,52.7 v19.56,59.05
  Bottom 1.27: U$2.15 20.19,50.8 19.56,51.44 v19.56,52.7 | v19.56,59.05 JP3.16
T3OUT_0
  Bottom 1.27: U$3.28 20.19,36.83 19.56,36.2 JP4.1
T3OUT_1
  Bottom 1.27: JP4.2 U$3.1
T3OUT_2
  Bottom 1.27: JP4.3 U$3.2
T3OUT_3
  Bottom 1.27: JP4.4 U$3.3
T3OUT_4
  Bottom 1.27: JP4.5 U$3.4
T3OUT_5
  Bottom 1.27: JP4.6 U$3.5
T3OUT_6
  Bottom 1.27: JP4.7 U$3.6
T3OUT_7
  Bottom 1.27: JP4.8 U$3.7
T3OUT_8
  Bottom 1.27: JP4.9 U$3.8
T3OUT_9
  Bottom 1.27: JP4.10 U$3.9
T3OUT_10
  Bottom 1.27: JP4.11 U$3.10
T3OUT_11
  Bottom 1.27: JP4.12 U$3.11
T3OUT_12
  Bottom 1.27: JP4.13 U$3.12
T3OUT_13
  Bottom 1.27: JP4.14 U$3.13
T3OUT_14
  Bottom 1.27: JP4.15 U$3.14
T3OUT_15  (via drill 0.8)
  Top 0.813: v57.66,36.83 v57.66,28.58
  Bottom 0.813: U$3.15 v57.66,36.83 | v57.66,28.58 JP4.16
T4OUT0
  Bottom 0.813: U$5.28 62.74,36.83 61.47,35.56 JP8.1
T4OUT1
  Bottom 1.27: JP8.2 U$5.1
T4OUT2
  Bottom 1.27: JP8.3 U$5.2
T4OUT3
  Bottom 1.27: JP8.4 U$5.3
T4OUT4
  Bottom 1.27: JP8.5 U$5.4
T4OUT5
  Bottom 1.27: JP8.6 U$5.5
T4OUT6
  Bottom 1.27: JP8.7 U$5.6
T4OUT7
  Bottom 1.27: JP8.8 U$5.7
T4OUT8
  Bottom 1.27: JP8.9 U$5.8
T4OUT9
  Bottom 1.27: JP8.10 U$5.9
T4OUT10
  Bottom 1.27: JP8.11 U$5.10
T4OUT11
  Bottom 1.27: JP8.12 U$5.11
T4OUT12
  Bottom 1.27: JP8.13 U$5.12
T4OUT13
  Bottom 1.27: JP8.14 U$5.13
T4OUT14
  Bottom 1.27: JP8.15 U$5.14
T4OUT15  (via drill 0.8)
  Top 0.813: v99.57,29.21 v99.57,34.92
  Bottom 0.813: JP8.16 v99.57,29.21 | v99.57,34.92 99.57,36.2 98.93,36.83 U$5.15
T5OUT0  (via drill 0.8)
  Top 0.813: v113.54,11.43 v121.16,11.43
  Bottom 1.27: v113.54,11.43 U$6.28 | v121.16,11.43 JP9.1
T5OUT1
  Bottom 1.27: JP9.2 U$6.1
T5OUT2
  Bottom 1.27: JP9.3 U$6.2
T5OUT3
  Bottom 1.27: JP9.4 U$6.3
T5OUT4
  Bottom 1.27: JP9.5 U$6.4
T5OUT5
  Bottom 1.27: JP9.6 U$6.5
T5OUT6
  Bottom 1.27: JP9.7 U$6.6
T5OUT7
  Bottom 1.27: JP9.8 U$6.7
T5OUT8
  Bottom 1.27: JP9.9 U$6.8
T5OUT9
  Bottom 1.27: JP9.10 U$6.9
T5OUT10
  Bottom 1.27: JP9.11 U$6.10
T5OUT11
  Bottom 1.27: JP9.12 U$6.11
T5OUT12
  Bottom 1.27: JP9.13 U$6.12
T5OUT13
  Bottom 1.27: JP9.14 U$6.13
T5OUT14
  Bottom 1.27: JP9.15 U$6.14
T5OUT15  (via drill 0.8)
  Top 0.813: v113.54,49.21 121.61,49.21 v121.79,49.15
  Bottom 1.27: U$6.15 v113.54,49.21 | JP9.16 122.17,49.53 v121.79,49.15
T6OUT0  (via drill 0.8)
  Top 0.813: v99.57,9.52 v99.57,17.15
  Bottom 1.27: U$7.28 v99.57,9.52 | v99.57,17.15 JP10.1
T6OUT1
  Bottom 1.27: JP10.2 U$7.1
T6OUT2
  Bottom 1.27: JP10.3 U$7.2
T6OUT3
  Bottom 1.27: JP10.4 U$7.3
T6OUT4
  Bottom 1.27: JP10.5 U$7.4
T6OUT5
  Bottom 1.27: JP10.6 U$7.5
T6OUT6
  Bottom 1.27: JP10.7 U$7.6
T6OUT7
  Bottom 1.27: JP10.8 U$7.7
T6OUT8
  Bottom 1.27: JP10.9 U$7.8
T6OUT9
  Bottom 1.27: JP10.10 U$7.9
T6OUT10
  Bottom 1.27: JP10.11 U$7.10
T6OUT11
  Bottom 1.27: JP10.12 U$7.11
T6OUT12
  Bottom 1.27: JP10.13 U$7.12
T6OUT13
  Bottom 1.27: JP10.14 U$7.13
T6OUT14
  Bottom 1.27: JP10.15 U$7.14
T6OUT15  (via drill 0.8)
  Top 0.813: v61.47,9.52 v61.47,17.78
  Bottom 1.27: v61.47,17.78 JP10.16 | v61.47,9.52 U$7.15
T7OUT0  (via drill 0.8)
  Top 0.813: v57.66,9.52 v57.66,17.78
  Bottom 0.813: 57.66,19.69 JP11.1
  Bottom 1.27: U$8.28 v57.66,9.52 | v57.66,17.78 57.66,19.69
T7OUT1
  Bottom 1.27: JP11.2 U$8.1
T7OUT2
  Bottom 1.27: JP11.3 U$8.2
T7OUT3
  Bottom 1.27: JP11.4 U$8.3
T7OUT4
  Bottom 1.27: JP11.5 U$8.4
T7OUT5
  Bottom 1.27: JP11.6 U$8.5
T7OUT6
  Bottom 1.27: JP11.7 U$8.6
T7OUT7
  Bottom 1.27: JP11.8 U$8.7
T7OUT8
  Bottom 1.27: JP11.9 U$8.8
T7OUT9
  Bottom 1.27: JP11.10 U$8.9
T7OUT10
  Bottom 1.27: JP11.11 U$8.10
T7OUT11
  Bottom 1.27: JP11.12 U$8.11
T7OUT12
  Bottom 1.27: JP11.13 U$8.12
T7OUT13
  Bottom 1.27: JP11.14 U$8.13
T7OUT14
  Bottom 1.27: JP11.15 U$8.14
T7OUT15
  Bottom 1.27: U$8.15 20.83,9.52 19.56,10.8 JP11.16
TX  (via drill 0.8)  (2 unrouted)
  Bottom 1.016: SV1.1 v62.61,76.2
  Bottom 1.27: v89.15,73.91 MODUL1.J1.1
VCC  (via drill 0.8)  (4 unrouted)
  Top 0.813: v125.98,96.52 v112.65,96.52 | v110.62,96.52 v92.96,96.52 | v90.42,96.52 v84.07,96.52 | v65.02,86.36 v65.02,99.06
  Bottom 0.813: 37.34,47.62 C11.2 | v65.02,99.06 68.83,99.06 | 68.83,99.06 69.15,99.38 | 70.1,100.33 R1.2 | 77.72,99.06 78.04,98.74 | R5.2 68.83,99.06 | 80.52,14.61 105.28,14.61 110.36,9.52 113.54,9.52 | 80.52,14.61 C12.2 38.61,14.61 | 38.61,14.61 33.53,14.61 32.26,13.34 U$8.19 | U$3.19 44.96,34.92 43.69,33.66 41.15,33.66 39.88,34.92 U$3.21 C5.2 39.88,43.81 37.34,46.36 C11.2 | C11.2 U$2.21 37.34,54.61 38.61,55.88 | 33.53,55.88 32.26,54.61 U$2.19 | 33.53,55.88 38.61,55.88 | 38.61,55.88 76.07,55.88 | 80.52,55.88 76.07,55.88 | U$1.19 74.17,53.98 76.07,55.88 | 80.52,55.88 79.25,54.61 U$1.21 C4.2 79.25,46.36 81.79,43.81 C14.2 U$5.21 81.79,34.92 83.06,33.66 85.6,33.66 86.87,34.92 U$5.19 | 80.52,55.88 100.2,55.88 103.38,59.05 C2.+ 121.03,59.05 121.79,58.29 C13.2 ARDUINO2LEDDRIVER.7 121.79,51.69 118.62,48.51 118.62,38.1 117.03,36.51 | 117.03,36.51 116.71,36.2 116.08,36.83 U$6.19 | 117.03,36.51 117.03,30.99 | 117.03,30.99 117.03,11.11 | 117.03,11.11 115.44,9.52 113.54,9.52 | 113.54,9.52 C15.+ | 80.52,14.61 79.25,13.34 U$7.21 79.25,8.26 77.98,6.98 75.44,6.98 74.17,8.26 U$7.19 | 38.61,14.61 37.34,13.34 U$8.21 C3.2 | 117.03,11.11 119,9.14 C16.+ | 33.53,55.88 18.67,55.88 17.91,55.12 17.91,48.39 18.67,47.62 C18.+ | R16.1 109.5,97.69 109.47,97.66 | 117.03,30.99 116.27,31.75 U$6.21
  Bottom 1.27: 70.1,77.47 R9.2 | 58.04,90.17 58.04,87.63 59.31,86.36 | 58.04,90.17 59.31,91.44 SV5.2 | v65.02,99.06 R5.2 | 69.15,99.38 70.1,100.33 | R1.2 70.1,102.87 Q4.3 | R5.2 73.91,102.87 Q3.3 | R5.2 77.72,99.06 | 78.04,98.74 80.26,96.52 D1.A v84.07,96.52 | v90.42,96.52 v92.96,96.52 92.96,97.79 91.69,99.06 R6.1 86.61,100.33 Q2.3 | v112.65,96.52 v110.62,96.52 109.47,97.66 Q5.3 | Q1.3 104.39,102.87 107.57,99.69 R7.1 R16.1 | 125.98,99.06 Q6.3 | v125.98,96.52 125.98,99.06 | R15.2 125.98,99.06 | 59.31,86.36 v65.02,86.36 65.02,76.2 66.93,74.3 C6.1 78.36,74.3 79.63,73.03 C1.+ 82.17,71.75 83.44,70.48 108.84,70.48 LEDDRIVER2ARDUINO.7 | S1.1 5.71,36.07 8.89,39.24 SV4.2 | SV1.4 59.82,85.85 59.31,86.36 | 58.04,90.17 58.04,95.63 C17.+ | C10.2 70.1,77.47 | 70.1,77.47 IC1.1

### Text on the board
Top: HC- 05
Dimension: IN + - | NANO | IN + -
tPlace: RX TX - +
tValues: + - GSC XL BL SIN SCL | 0 | 0 | SCL SIN BL XL GSC - + | 0 | 0 | 0 | 0 | 0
